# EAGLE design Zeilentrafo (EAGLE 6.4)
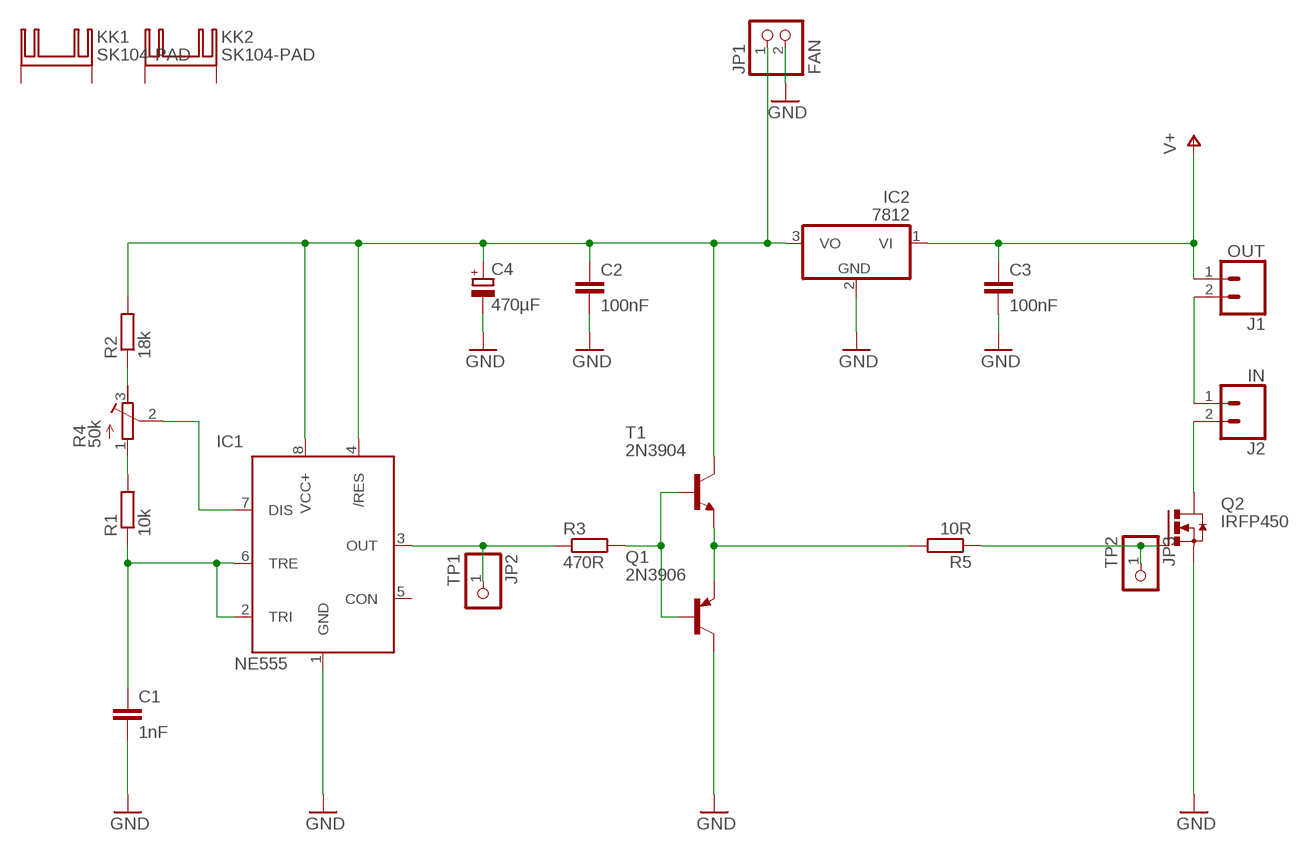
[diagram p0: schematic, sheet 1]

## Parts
C1  1nF  C-EU050-024X044  [C050-024X044]
C2  100nF  C-EU050-024X044  [C050-024X044]
C3  100nF  C-EU050-024X044  [C050-024X044]
C4  470µF  CPOL-EUE5-10.5  [E5-10,5]
IC1  NE555  [DIL-08]
IC2  7812  7812TV  [TO220V]
J1  OUT  CONN_025MM  [SCREWTERMINAL-5MM-2]
J2  IN  CONN_025MM  [SCREWTERMINAL-5MM-2]
JP1  FAN  PINHD-1X2  [1X02]
JP2  TP1  PINHD-1X1  [1X01]
JP3  TP2  PINHD-1X1  [1X01]
KK1  SK104-PAD  [SK104-PAD]
KK2  SK104-PAD  [SK104-PAD]
Q1  2N3906  [TO92]
Q2  IRFP450  IRFP240  [TO247BV]
R1  10k  R-EU_0207/5V  [0207/5V]
R2  18k  R-EU_0207/12  [0207/12]
R3  470R  R-EU_0207/12  [0207/12]
R4  50k  R-TRIMM3296Y  [RTRIM3296Y]
R5  10R  R-EU_0207/12  [0207/12]
T1  2N3904  [TO92]

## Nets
GND: C1.2 C2.2 C3.2 C4.- IC1.1(GND) IC2.2(GND) JP1.2 Q1.1(C) Q2.S
N$1: C1.1 IC1.2(TRI) IC1.6(TRE) R1.1
N$2: IC1.7(DIS) R4.2(S)
N$3: R1.2 R4.1(A)
N$4: R2.1 R4.3(E)
N$5: C2.1 C4.+ IC1.4(/RES) IC1.8(VCC+) IC2.3(VO) JP1.1 R2.2 T1.1(C)
N$6: JP3.1 Q2.G R5.1
N$7: IC1.3(OUT) JP2.1 R3.1
N$8: Q1.2(B) R3.2 T1.2(B)
N$9: Q1.3(E) R5.2 T1.3(E)
N$10: J1.2 J2.1
N$13: J2.2 Q2.D
V+: C3.1 IC2.1(VI) J1.1
Unconnected: IC1.5(CON) KK1.K1(K) KK1.K2(K) KK2.K1(K) KK2.K2(K)

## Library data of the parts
C1-C3 = rcl_custom:C-EU: CAPACITOR, European symbol
C4 = rcl_custom:CPOL-EU: POLARIZED CAPACITOR, European symbol
IC1 = st-microelectronics_custom:NE555: General purpose bipolar Timer; MF: Arrow Electronics; MPN: NE555N; OC_FARNELL: 1467742; OC_NEWARK: 89K1486
IC2 = linear:78*: Positive VOLTAGE REGULATOR Source: http://cache.national.com/ds/LM/LM78L05.pdf http://www.fairchildsemi.com/ds/LM/LM7805.pdf
J1 J2 = SparkFun-Connectors:CONN_02: Multi connection point. Often used as Generic Header-pin footprint for 0.1 inch spaced/style header connections; SF_SKU: PRT-08432
JP1 = pinhead:PINHD-1X2: PIN HEADER
JP2 JP3 = pinhead:PINHD-1X1: PIN HEADER
KK1 KK2 = heatsink_custom:SK104-PAD: HEATSINK
Q1 = transistor-pnp:2N3906: PNP Transistor
Q2 = transistor-power:IRFP240: HEXFET Power MosFet Source: http://www.irf.com/
R1 = rcl:R-EU_: RESISTOR, European symbol
R2 R3 R5 = rcl_custom:R-EU_: RESISTOR, European symbol
R4 = rcl:R-TRIMM: Trimm resistor
T1 = transistor:2N3904: NPN TRANSISTOR

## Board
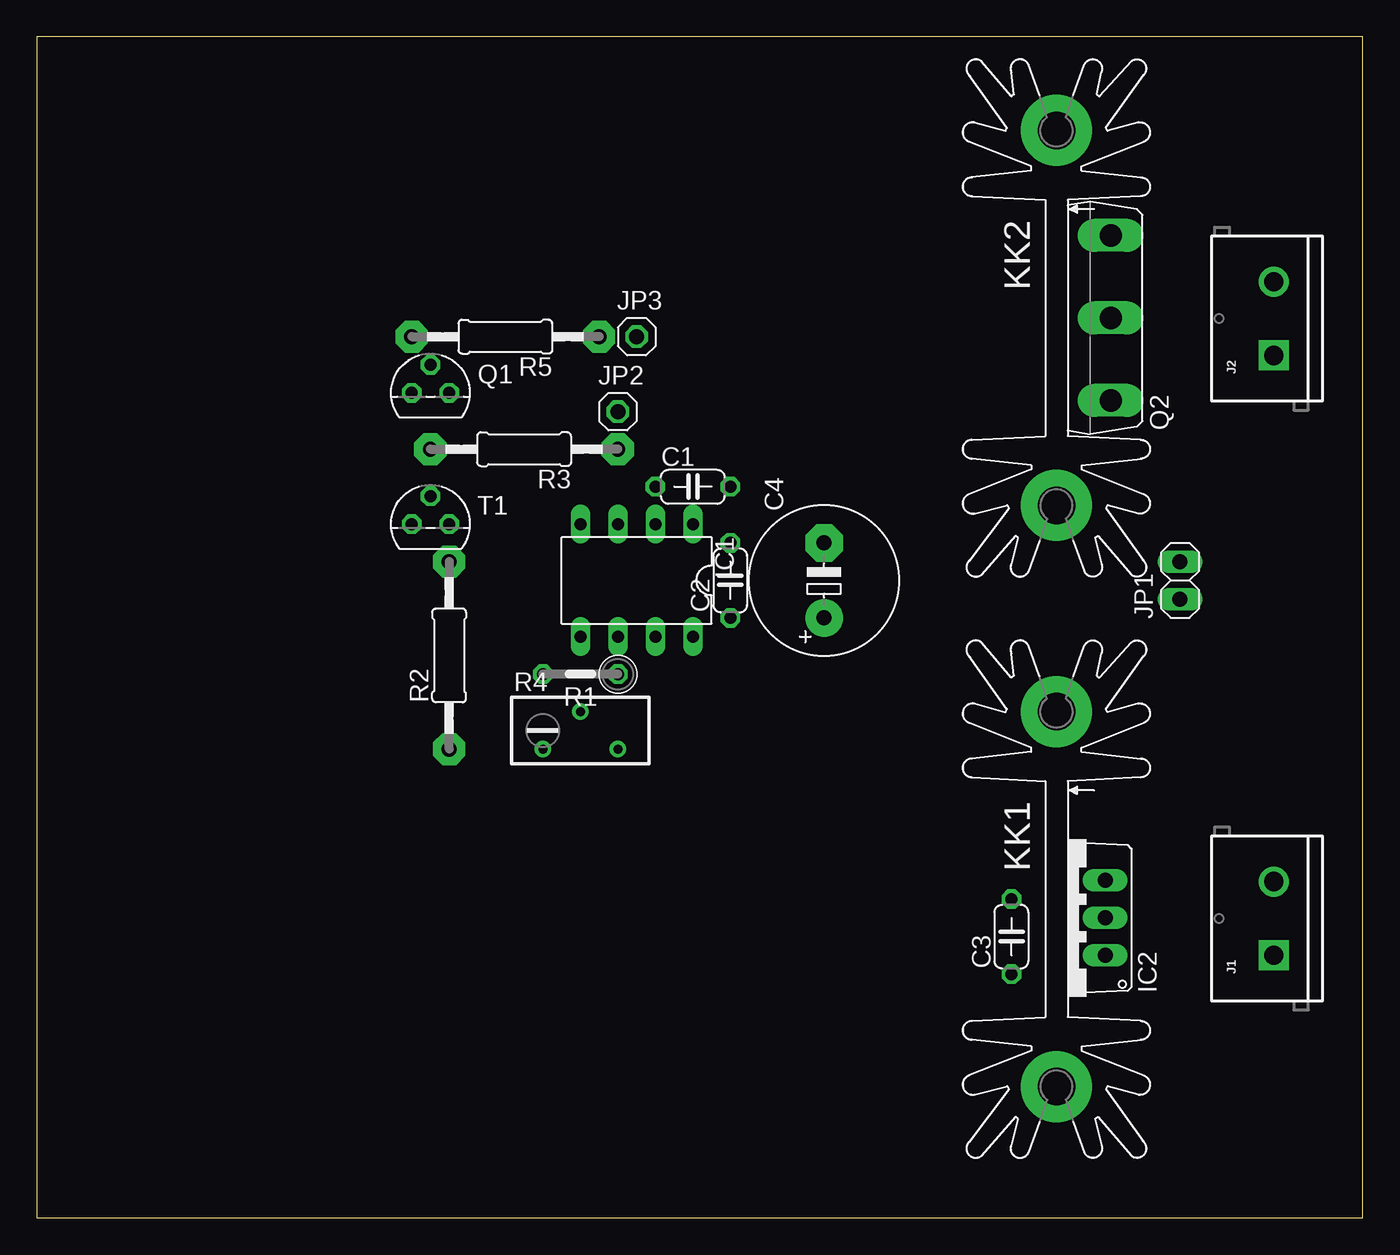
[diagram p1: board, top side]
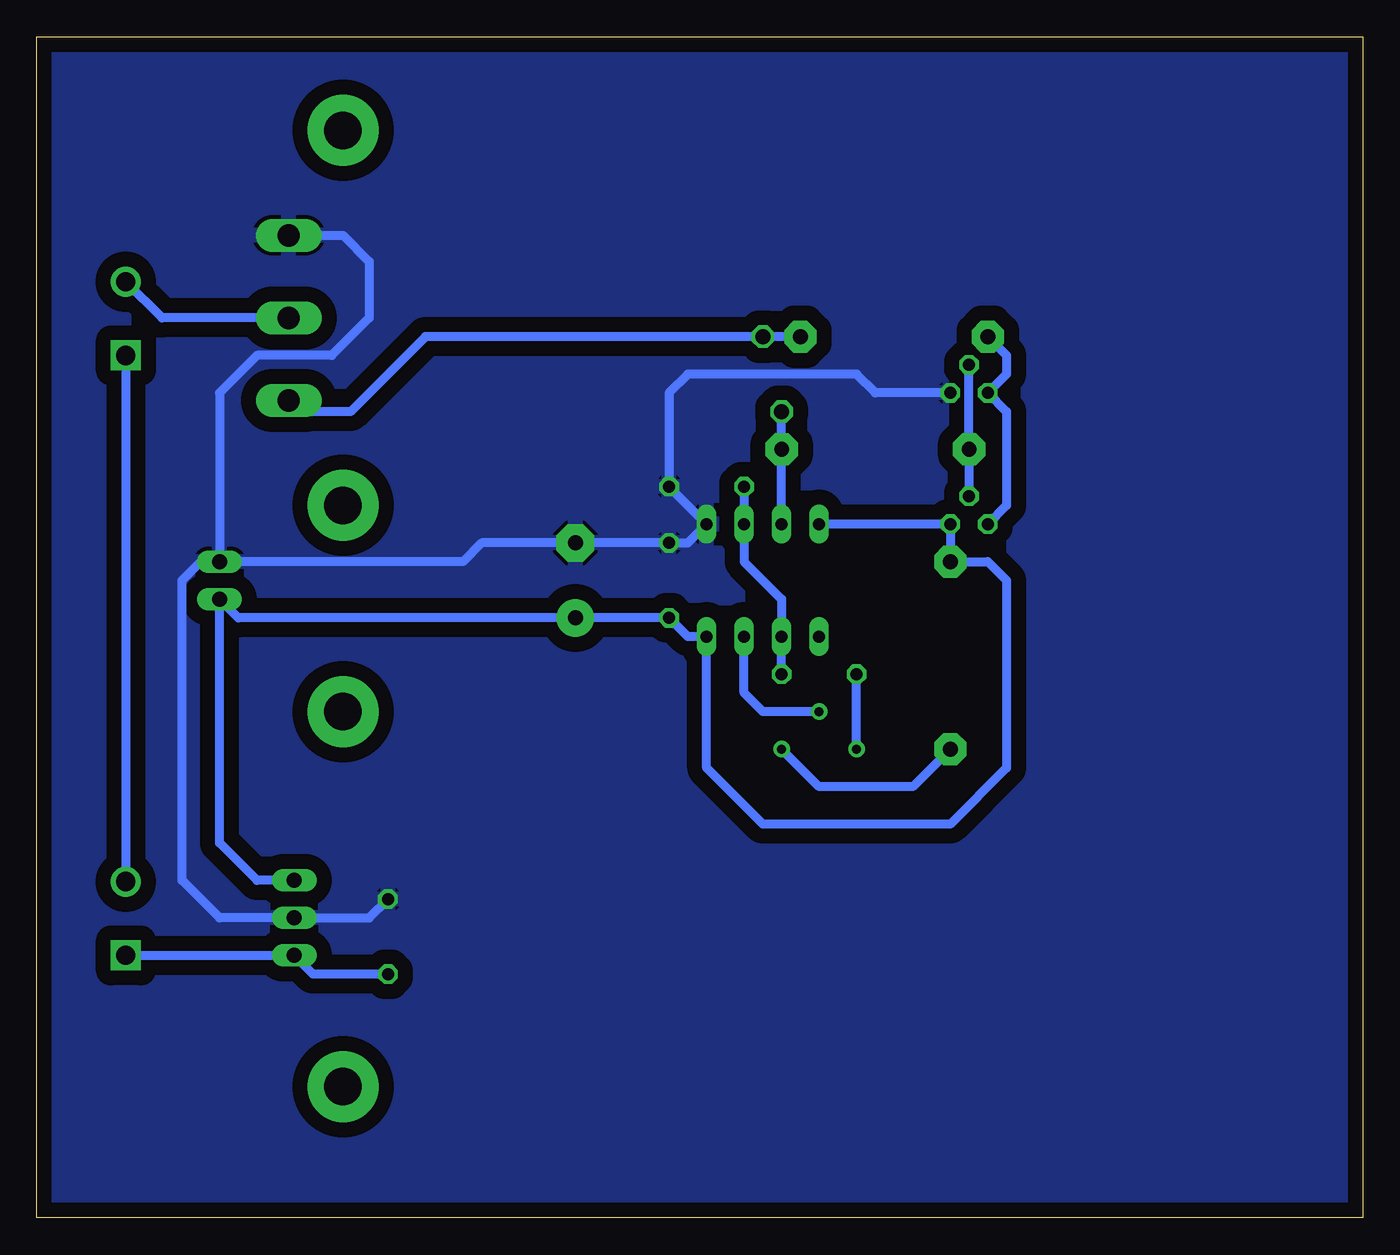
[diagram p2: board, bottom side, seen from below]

Size 89.84 x 80 mm. Coordinates in mm from the lower left corner, seen from the top.
Outline: 0,0 89.84,0 89.84,80 0,80 0,0
Copper layers (1*16): Top 0.035mm / dielectric 1.5mm / Bottom 0.035mm
Design rules "default *": minimum track width 25mil, minimum drill 0.35mm, track to track 12mil, track to pad 12mil, pad to pad 6mil, via to via 6mil, smd to smd 6mil, copper to edge 40mil, drill to drill 6mil, minimum pad ring 10mil, minimum via ring 8mil, stop-mask expansion 4mil, vias tented up to drill 0mil, thermal gap 10mil

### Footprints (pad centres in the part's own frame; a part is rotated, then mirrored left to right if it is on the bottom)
C050-024X044 = drill 0.813 octagon: 1 -2.54,0; 2 2.54,0
E5-10,5 = drill 1.016 pad 2.54: + -2.54,0 | drill 1.016 pad 2.54 octagon: - 2.54,0
DIL-08 = drill 0.813 long: 1 -3.81,-3.81; 2 -1.27,-3.81; 3 1.27,-3.81; 4 3.81,-3.81; 5 3.81,3.81; 6 1.27,3.81; 7 -1.27,3.81; 8 -3.81,3.81
TO220V = drill 1.016 long: 1 -2.54,-2.54; 2 0,-2.54; 3 2.54,-2.54
SCREWTERMINAL-5MM-2 = drill 1.3 pad 2.032 square: 1 0,0 | drill 1.3 pad 2.032: 2 5,0
1X02 = drill 1.016 long: 1 -1.27,0; 2 1.27,0
1X01 = drill 1.016 octagon: 1 0,0
SK104-PAD = drill 2.54 pad 4.81: K1 -12.7,-0.762; K2 12.7,-0.762
TO92 = drill 0.813 octagon: 1 1.27,0; 2 0,1.905; 3 -1.27,0
TO247BV = drill 1.499 long: D 0,-2.921; G -5.588,-2.921; S 5.588,-2.921
0207/5V = drill 0.813 octagon: 1 -2.54,0; 2 2.54,0
0207/12 = drill 1 pad 2.184 octagon: 1 -6.35,0; 2 6.35,0
RTRIM3296Y = drill 0.61: 1 1.27,-2.54; 2 -1.27,0; 3 1.27,2.54

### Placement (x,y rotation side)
C1  44.45,49.53 0 top
C2  46.99,43.18 90 top
C3  66.04,19.05 90 top
C4  53.34,43.18 90 top
IC1  40.64,43.18 180 top
IC2  69.85,20.32 90 top
J1  83.82,17.78 90 top
J2  83.82,58.42 90 top
JP1  77.47,43.18 90 top
JP2  39.37,54.61 0 top
JP3  40.64,59.69 0 top
KK1  69.85,21.59 270 top
KK2  69.85,60.96 270 top
Q1  26.67,55.88 0 top
Q2  69.85,60.96 90 top
R1  36.83,36.83 180 top
R2  27.94,38.1 90 top
R3  33.02,52.07 180 top
R4  36.83,33.02 270 top
R5  31.75,59.69 180 top
T1  26.67,46.99 0 top

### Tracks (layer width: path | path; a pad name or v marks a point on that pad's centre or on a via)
GND
  Bottom 0.6: C3.2 67.31,20.32 IC2.2 77.47,20.32 80.01,22.86 80.01,43.18 78.74,44.45 JP1.2 | Q2.S 69.09,66.55 67.31,64.77 67.31,60.96 69.85,58.42 74.93,58.42 77.47,55.88 JP1.2 | JP1.2 60.96,44.45 59.69,45.72 C4.- C2.2 45.72,45.72 IC1.1 C1.2 46.99,55.88 45.72,57.15 34.29,57.15 33.02,55.88 Q1.1
  pour Bottom (isolate 1.016): 0,80.01 90.17,80.01 90.17,0 0,0
N$1
  Bottom 0.6: C1.1 IC1.2 41.91,44.45 39.37,41.91 IC1.6 R1.1
N$2
  Bottom 0.6: R4.2 40.64,34.29 41.91,35.56 IC1.7
N$3
  Bottom 0.6: R4.1 R1.2
N$4
  Bottom 0.6: R2.1 30.48,29.21 36.83,29.21 R4.3
N$5
  Bottom 0.6: IC1.4 T1.1 R2.2 25.4,44.45 24.13,43.18 24.13,30.48 27.94,26.67 40.64,26.67 44.45,30.48 IC1.8 45.72,39.37 C2.1 C4.+ 76.2,40.64 JP1.1 77.47,25.4 74.93,22.86 IC2.3
N$6
  Bottom 0.6: JP3.1 R5.1 63.5,59.69 68.58,54.61 72.01,54.61 Q2.G
N$7
  Bottom 0.6: IC1.3 R3.1 JP2.1
N$8
  Bottom 0.6: Q1.2 R3.2 T1.2
N$9
  Bottom 0.6: R5.2 24.13,58.42 24.13,57.15 Q1.3 24.13,54.61 24.13,48.26 T1.3
N$10
  Bottom 0.6: J2.1 J1.2
N$13
  Bottom 0.6: Q2.D 81.36,60.96 J2.2
V+
  Bottom 0.6: J1.1 IC2.1 71.12,16.51 C3.1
